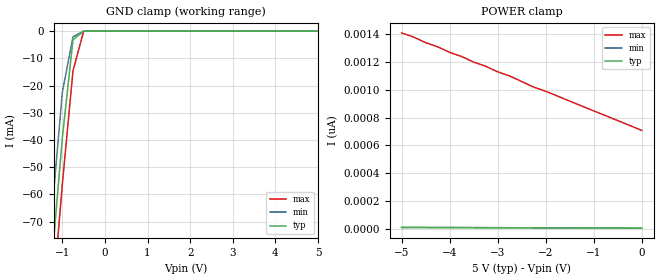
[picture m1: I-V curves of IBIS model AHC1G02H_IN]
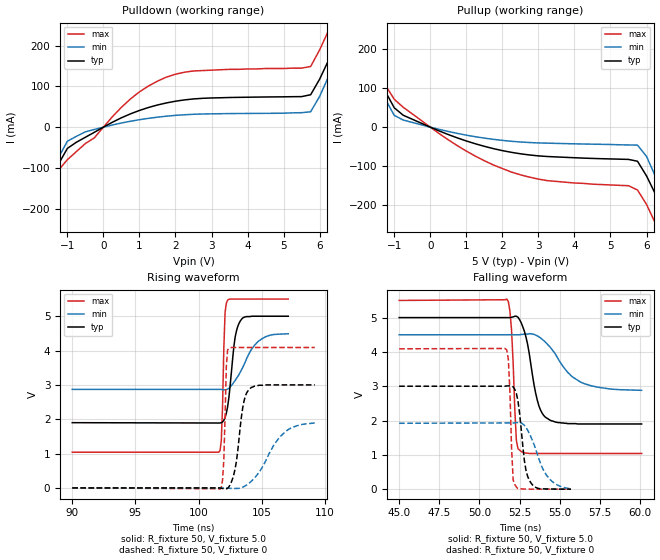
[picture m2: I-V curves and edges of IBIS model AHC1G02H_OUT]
| TEXAS INSTRUMENTS INCORPORATED
| Standard Linear and Logic Group
| IBIS Model of SN74AHC1G02H
| SINGLE 2-INPUT POSITIVE-NOR GATE
| CMPAK-5 5-pin (DCK) Package
[IBIS Ver]   2.1
[Comment Char]  |_char
[File name]   ul02_5c.ibs
[File Rev]   2.0
[Date]   April 17, 2000
[Source]   Data created from SPICE simulations at Hitachi,Ltd.
[Notes]   The following is an IBIS List for the AHC1G02H.
|   Please contact sllibis@ti.com with questions and
|   comments concerning SLL IBIS models.
[Disclaimer] Property of Texas Instruments Incorporated.  Unauthorized
   reproduction and/or distribution is strictly prohibited.
   This product is protected under copyright law.
   Created 2000, (C) Copyright 2000, Texas Instruments Inc.,
   All Rights Reserved.
   UNLESS THERE IS A SIGNED, WRITTEN AGREEMENT TO THE
   CONTRARY, TEXAS INSTRUMENTS () IS PROVIDING THE IBIS
   MODELS  AND WITHOUT ANY WARRANTY, EXPRESSED OR
   IMPLIED.  TI assumes no liability for:
   1) the accuracy of the IBIS models provided to your
   company;
   2) the proper functioning of these IBIS Models in your
   design or for any resulting applications; or
   3) infringement of patents, copyrights or intellectual
   property rights resulting from your use of these IBIS
   models.
   TI provides IBIS Models as a service to our customers.
   You and your company shall not distribute, sell or give
   these models to anyone else without prior written
   permission from TI.
   TI reserves the right to make changes to our products or
   to discontinue any semiconductor product or service
   without notice, and advises our customers to obtain the
   latest version of relevant information to verify, before
   placing orders, that the information being relied on is
   current.
   Please be aware that your receipt and use of the IBIS
   information provided shall serve as acceptance of these
   terms and conditions.  If you do not accept these terms,
   you should return or destroy the IBIS models and any
   other accompanying information immediately.
|   Component AHC1G02H
[Component]   AHC1G02H
[Manufacturer]   Hitachi, Ltd.
[Package]
|   typ   min   max
R_pkg   0.090   0.051   0.105
L_pkg   1.500nH   0.940nH   1.700nH
C_pkg   0.170pF   0.110pF   0.360pF
[Pin]   signal_name   model_name   R_pin   L_pin   C_pin
1   A   AHC1G02H_IN   0.098   1.590nH   0.110pF
2   B   AHC1G02H_IN   0.051   0.940nH   0.170pF
3   GND   GND   0.092   1.590nH   0.360pF
4   Y   AHC1G02H_OUT   0.105   1.700nH   0.110pF
5   VCC   POWER   0.104   1.690nH   0.110pF
| Models and submodels in the file (2): AHC1G02H_IN (Input), AHC1G02H_OUT (Output)
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|   Model AHC1G02H_IN
[Model]   AHC1G02H_IN
Model_type  Input
Polarity   Inverting
Vinl = 1.50
Vinh = 3.50
| variable   typ   min   max
C_comp   2.19pF   2.07pF   2.30pF
[Temperature Range]   25   85   -40
[Voltage Range]   5.0   4.5   5.5
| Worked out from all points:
|   GND clamp passes 1 mA (typ) near -0.58 V on its own axis
[GND Clamp]
|   Voltage   I(typ)   I(min)   I(max)
-5V       -823mA     -807mA     -840mA
-1.5V     -133mA     -115mA     -150mA
-1.25V    -85.2mA    -67.5mA    -103mA
-1V       -39.2mA    -22.5mA    -56.2mA
-750mV    -3.18mA    -2.09mA    -14.6mA
-500mV    -11.6uA    -2.99uA    -57.1uA
5V        5.34pA     5pA        708pA
[POWER Clamp]
|   Voltage   I(typ)   I(min)   I(max)
-5V       10.6pA     10pA       1.41nA
-4.75V    10.3pA     9.75pA     1.38nA
-4.5V     10pA       9.5pA      1.34nA
-4.25V    9.78pA     9.25pA     1.31nA
-4V       9.52pA     9pA        1.27nA
-3.75V    9.26pA     8.75pA     1.24nA
-3.5V     9pA        8.5pA      1.2nA
-3.25V    8.74pA     8.25pA     1.17nA
-2.75V    8.21pA     7.75pA     1.1nA
-2.25V    7.69pA     7.25pA     1.02nA
-2V       7.43pA     7pA        990pA
0V        5.34pA     5pA        708pA
|   Model AHC1G02H_OUT
[Model]   AHC1G02H_OUT
Model_type  Output
Polarity   Non-Inverting
Vmeas = 2.5
Cref = 15pf
| variable   typ   min   max
C_comp   4.52pF   4.32pF   4.72pF
[Temperature Range]   25   85   -40
[Voltage Range]   5.0   4.5   5.5
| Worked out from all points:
|   slope of the pulldown table from 0 to 0.75 V, typ, clamps not added: 23 ohm
|   slope of the pullup table from 0 to 0.75 V, typ, clamps not added: 27.3 ohm
|   rising waveform, R_fixture 50, V_fixture 5.0: 20-80 % time 533ps typ, 1.46ns min, 196ps max; typ from 1.9 V to 5 V
|   falling waveform, R_fixture 50, V_fixture 5.0: 20-80 % time 723ps typ, 1.69ns min, 243ps max; typ from 5 V to 1.9 V
|   falling waveform, R_fixture 50, V_fixture 0: 20-80 % time 433ps typ, 1.01ns min, 189ps max; typ from 3 V to 0 V
|   rising waveform, R_fixture 50, V_fixture 0: 20-80 % time 616ps typ, 1.88ns min, 182ps max; typ from 0 V to 3 V
[Pulldown]
|   Voltage   I(typ)   I(min)   I(max)
-5V       -826mA     -810mA     -842mA
-2.25V    -282mA     -267mA     -299mA
-2V       -234mA     -219mA     -250mA
-1.25V    -91.3mA    -75.2mA    -106mA
-1V       -52.3mA    -34.7mA    -80mA
750mV     32.6mA     14.5mA     69.2mA
1.75V     59.5mA     26.9mA     123mA
5.75V     79.6mA     37.8mA     149mA
6.25V     165mA      125mA      238mA
6.75V     261mA      217mA      336mA
7V        310mA      265mA      385mA
10V       906mA      861mA      980mA
[Pullup]
|   Voltage   I(typ)   I(min)   I(max)
-5V       828mA      811mA      845mA
-2.25V    284mA      267mA      301mA
-2V       235mA      218mA      252mA
-1V       49.6mA     30.1mA     71.4mA
750mV     -27.5mA    -16mA      -47.4mA
2.25V     -64.5mA    -36.2mA    -115mA
5.75V     -87.4mA    -46mA      -161mA
6V        -125mA     -75mA      -198mA
6.25V     -172mA     -127mA     -247mA
6.75V     -269mA     -224mA     -345mA
7V        -318mA     -273mA     -395mA
10V       -917mA     -874mA     -991mA
[Ramp]
| variable   typ   min   max
dV/dt_r   1.80E+00/6.10E-10   1.15E+00/1.92E-09   2.45E+00/1.80E-10
dV/dt_f   1.86E+00/7.20E-10   9.76E-01/1.69E-09   2.68E+00/2.40E-10
R_load = 50
[Rising Waveform]
R_fixture = 50
V_fixture = 5.0
V_fixture_min = 4.5
V_fixture_max = 5.5
|   Time   V(typ)   V(min)   V(max)
90ns      1.9V       2.87V      1.04V
101.6ns   1.89V      2.87V      1.04V
101.8ns   1.9V       2.87V      1.37V
101.9ns   1.92V      2.86V      2.38V
102.1ns   2.05V      2.86V      5.12V
102.3ns   2.36V      2.88V      5.47V
102.9ns   4.4V       3.13V      5.5V
103.3ns   4.86V      3.37V      5.5V
104.8ns   5V         4.29V      5.5V
107.1ns   5V         4.49V      5.5V
[Falling Waveform]
R_fixture = 50
V_fixture = 5.0
V_fixture_min = 4.5
V_fixture_max = 5.5
|   Time   V(typ)   V(min)   V(max)
45ns      5V         4.5V       5.5V
51.7ns    5V         4.5V       5.54V
51.9ns    5V         4.5V       5.18V
52ns      5.01V      4.5V       4.63V
52.3ns    5.04V      4.5V       1.42V
52.7ns    4.73V      4.51V      1.07V
53.6ns    2.6V       4.47V      1.04V
54.1ns    2.1V       4.29V      1.04V
56.3ns    1.9V       3.12V      1.04V
60.1ns    1.9V       2.88V      1.04V
[Falling Waveform]
R_fixture = 50
V_fixture = 0
|   Time   V(typ)   V(min)   V(max)
45ns      3V         1.92V      4.09V
51.6ns    3V         1.93V      4.1V
51.8ns    3.01V      1.93V      3.79V
52.1ns    2.98V      1.93V      264mV
52.2ns    2.91V      1.93V      136mV
52.4ns    2.57V      1.94V      14.5mV
52.8ns    830mV      1.86V      3.42mV
53.1ns    266mV      1.63V      910uV
54.2ns    5.89mV     393mV      -19uV
55.7ns    497uV      13.6mV     10uV
[Rising Waveform]
R_fixture = 50
V_fixture = 0
|   Time   V(typ)   V(min)   V(max)
90ns      0V         0V         0V
101.7ns   -2.19mV    411uV      -36.5mV
102ns     -22.6mV    63uV       821mV
102.2ns   -27mV      -4.92mV    3.54V
102.3ns   -10.8mV    -8mV       4.02V
102.9ns   566mV      -16.5mV    4.09V
103.5ns   2.34V      22.8mV     4.09V
104ns     2.87V      137mV      4.09V
106.7ns   3V         1.58V      4.09V
109.2ns   3V         1.89V      4.09V
